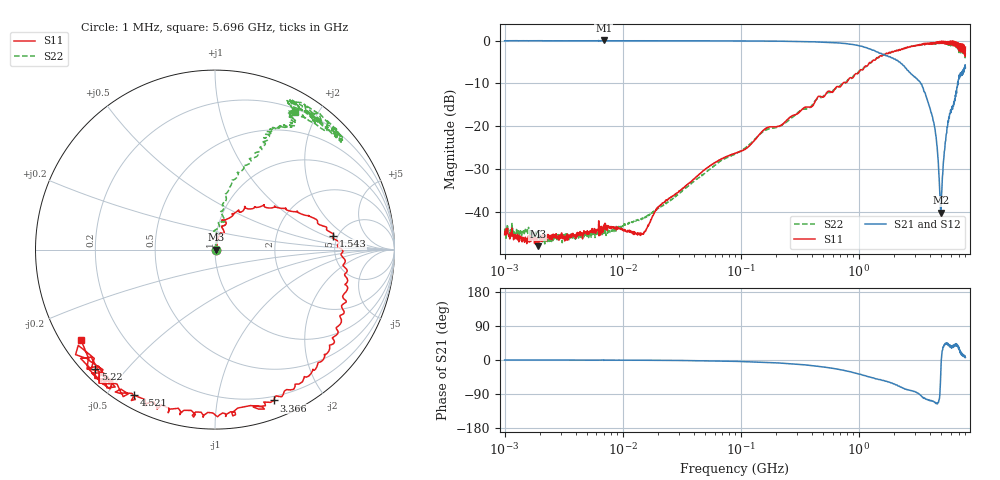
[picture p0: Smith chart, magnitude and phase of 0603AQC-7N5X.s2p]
!s-Parameter Generated by FASTRON Sdn. Bhd.
!FASTRON P/N : 0603AQC-7N5X
!Keysight Technologies: E5071C_MY46733604_B.14.02
!Date: Thu Jun 25 13:50:57 2026
!Version  :Rev00  Thu Jun 25 13:50:57 2026
!Data & Calibration Information:
!Freq  S11:SOLT2(ON)  S21:SOLT2(ON)  S12:SOLT2(ON)  S22:SOLT2(ON)
!PortZ  Port1:50+j0  Port2:50+j0
!When reading reference impedance value at option line is always used.
! Remarks : This data is being provided solely for informational purposes.
# Hz S dB R 50
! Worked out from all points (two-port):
!   1601 points, 1 MHz to 8 GHz, reference 50 ohm
!   highest |S21| = 0.02 dB at 6.912 MHz (marker M1); lowest = -40.1 dB at 4.94 GHz (marker M2)
!   |S21| within 3 dB of the highest: start of sweep to 1.544 GHz
!   lowest |S11| = -47.9 dB at 1.91 MHz (marker M3), VSWR 1.01, Z = 50.4 + j0.0162 ohm
!   |S11| at or under -10 dB: start of sweep to 731.1 MHz
!   |S22| runs from -47.4 to -0.4 dB; largest |S21 - S12| = 0.022
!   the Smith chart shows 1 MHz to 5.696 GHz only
!   S11 on the Smith chart (normalised r, x): 1 MHz: 1.01, -0.00; 1.543 GHz: 4.59, +1.25; 3.366 GHz: 0.16, -1.45; 4.521 GHz: 0.05, -0.59; 5.22 GHz: 0.03, -0.41; 5.696 GHz: 0.06, -0.30
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1000000  -45.20 -0.5  -0.05 -0.1  -0.06 -0.0  -43.90 2.6
1909681  -47.90 2.3  -0.06 -0.2  -0.06 -0.1  -46.00 5.1
4479405  -44.80 19.3  -0.05 -0.3  -0.06 -0.2  -45.80 25.4
6911657  -43.00 13.5  0.02 -0.9  -0.15 -0.3  -43.20 24.6
1.449233e7  -45.00 34.3  -0.05 -0.6  -0.06 -0.7  -41.40 45.6
2.00676e7  -38.90 45.5  -0.06 -0.9  -0.07 -0.8  -39.10 67.2
8.994653e7  -26.30 81.1  -0.09 -3.5  -0.09 -3.5  -26.40 74.1
4.006501e8  -15.40 74.5  -0.27 -14.8  -0.27 -14.8  -15.10 72.6
9.798081e8  -7.72 35.5  -1.13 -36.3  -1.14 -36.4  -7.55 73.2
1.542898e9  -3.56 6.6  -2.98 -52.5  -2.99 -52.7  -3.70 66.5
1.7949e9  -2.88 -3.7  -3.77 -58.1  -3.79 -58.3  -2.81 64.8
2.589603e9  -1.50 -37.7  -6.93 -78.2  -6.97 -78.3  -1.54 58.6
3.365624e9  -0.90 -68.7  -10.10 -93.9  -10.10 -93.9  -0.96 55.9
4.075033e9  -0.53 -97.3  -16.60 -107.0  -16.60 -108.0  -0.64 54.4
4.520586e9  -0.65 -119.0  -22.50 -115.0  -22.50 -115.0  -0.80 48.2
4.940464e9  -0.21 -131.0  -40.10 -40.8  -40.10 -40.8  -0.56 40.7
5.220382e9  -0.51 -135.0  -28.20 34.0  -28.20 33.7  -0.65 50.1
5.696244e9  -0.91 -146.0  -18.70 40.9  -18.70 40.7  -1.05 59.9
6.110812e9  -0.45 -161.0  -16.10 31.1  -16.10 30.8  -0.96 48.0
6.65058e9  -0.72 -152.0  -12.60 43.2  -12.50 42.7  -0.98 76.2
7.383122e9  -1.66 158.0  -7.73 13.8  -7.74 13.0  -2.35 54.1
8e9  -1.53 149.0  -6.32 6.3  -6.35 5.6  -2.68 63.7
